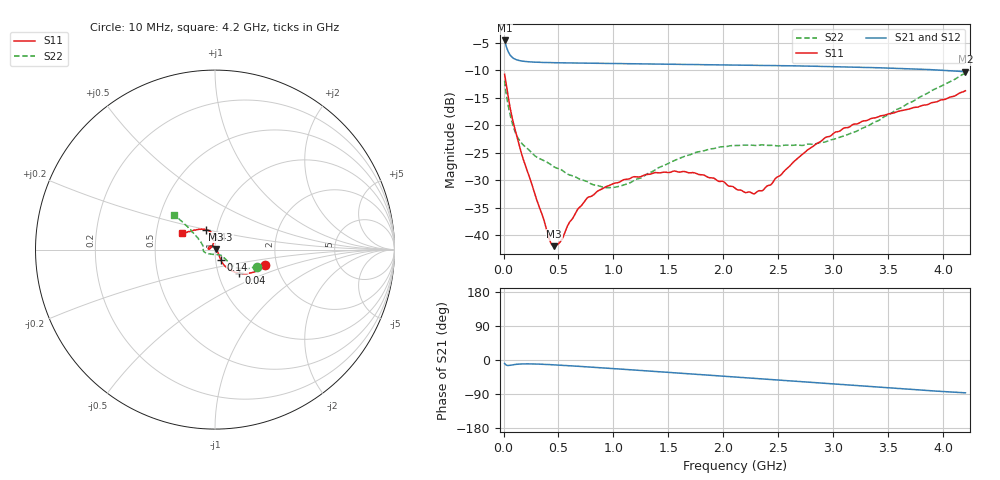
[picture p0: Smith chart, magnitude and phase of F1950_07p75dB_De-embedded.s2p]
! Integrated Device Technology
! Corporate Headquarters
! 6024 Silver Creek Valley Road
! San Jose, CA 95138  USA
! Phone:  1-408-284-8200
! Toll Free:  1-800-223-1366
! Webpage:  http://www.idt.com/
! Timing and RF Division
! 515 Groton Road, Suite 102
! Westford, MA 01886-6024
! Device:  F1950
! Description: 7-bit 0.25 dB Digital Step Attenuator
! Frequency:  150.0 -  4000.00 MHz
! Package:  4x4 mm Thin QFN Plastic Package: 24 pin
! Ports:  2 RF, 12 DC
!  Pin  1  = D0
!  Pin  2  = VDD
!  Pin  3  = Vmode
!  Pin  4  = GND
!  Pin  5  = RF1  =  Port 1
!  Pin  6  = GND
!  Pin  7  = GND
!  Pin  8  = GND
!  Pin  9  = GND
!  Pin 10  = GND
!  Pin 11  = GND
!  Pin 12  = GND
!  Pin 13  = GND
!  Pin 14  = RF2  =  Port 2
!  Pin 15  = GND
!  Pin 16  = LE
!  Pin 17  = CLK
!  Pin 18  = DATE
!  Pin 19  = D6
!  Pin 20  = D5
!  Pin 21  = D4
!  Pin 22  = D3
!  Pin 23  = D2
!  Pin 24  = D1
! State:  31
! Atten State:  7.75 dB
! Voltage:  +5.00 Volts
! Current:  Not Measured mA
! Data:  The device was measured on a the F195X evaluation board which has
!  individual transmission lines to the RF pins.  Data was collected
!  using a calibrated network analyzer.  The evaluation board was
!  de-embedded using a TRL calibration technique.
!  The reference plane is the edge of the package pin.
! Misc:  Board 2019
!  Action Tracker AT0250
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# GHz S dB R 50
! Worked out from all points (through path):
!   420 points, 10 MHz to 4.2 GHz, reference 50 ohm
!   highest |S21| = -4.56 dB at 10 MHz (marker M1); lowest = -10.3 dB at 4.2 GHz (marker M2)
!   group delay of S21, straight-line fit = 54.5 ps
!   lowest |S11| = -42.0 dB at 460 MHz (marker M3), VSWR 1.02, Z = 50.7 + j0.358 ohm
!   |S11| at or under -10 dB: start of sweep to end of sweep
!   |S22| runs from -31.3 to -10.5 dB; largest |S21 - S12| = 0.00048
!   S11 on the Smith chart (normalised r, x): 10 MHz: 1.73, -0.33; 40 MHz: 1.26, -0.35; 140 MHz: 1.06, -0.13; 3.43 GHz: 0.88, +0.20; 4.2 GHz: 0.68, +0.13
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0.01  -10.72 -17.3  -4.56 -9.3  -4.56 -9.3  -11.88 -21.8
0.04  -14.47 -44.4  -6.47 -14.4  -6.47 -14.4  -16.12 -40.3
0.09  -19.58 -59.2  -7.80 -12.4  -7.80 -12.4  -20.34 -43.0
0.14  -23.43 -60.8  -8.20 -10.8  -8.20 -10.8  -22.57 -42.1
0.29  -32.81 -46.7  -8.51 -10.6  -8.51 -10.6  -25.61 -42.1
0.41  -40.27 -8.7  -8.59 -12.0  -8.59 -12.0  -26.86 -43.5
0.46  -41.97 26.3  -8.61 -12.8  -8.61 -12.8  -27.55 -45.9
0.52  -41.07 66.0  -8.63 -13.8  -8.63 -13.8  -28.01 -48.2
0.59  -37.98 91.3  -8.65 -15.0  -8.65 -15.0  -28.93 -51.9
0.71  -34.56 111.1  -8.68 -17.2  -8.68 -17.2  -29.90 -61.3
0.86  -31.90 125.4  -8.72 -20.0  -8.72 -20.0  -30.96 -77.9
1.01  -30.52 136.3  -8.76 -22.9  -8.76 -22.9  -31.26 -99.6
1.41  -28.63 162.3  -8.85 -30.8  -8.85 -30.8  -27.70 -145.4
1.74  -28.64 174.6  -8.93 -37.4  -8.93 -37.5  -24.98 -162.4
2.11  -31.49 164.7  -9.03 -45.0  -9.03 -45.0  -23.69 -173.5
2.27  -32.44 141.0  -9.07 -48.3  -9.07 -48.3  -23.63 -177.1
2.36  -31.79 125.6  -9.10 -50.1  -9.10 -50.1  -23.55 -179.4
2.81  -23.89 95.5  -9.25 -59.4  -9.24 -59.4  -23.46 166.0
3.09  -20.55 100.8  -9.36 -65.2  -9.35 -65.2  -21.97 156.6
3.43  -18.28 114.1  -9.54 -72.2  -9.54 -72.2  -18.88 146.0
3.51  -17.87 117.7  -9.58 -73.8  -9.58 -73.9  -18.01 144.7
4.2  -13.71 153.9  -10.26 -86.6  -10.26 -86.7  -10.51 139.3
